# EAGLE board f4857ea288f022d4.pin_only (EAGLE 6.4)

Size 68.58 x 53.34 mm. Coordinates in mm from the lower left corner, seen from the top.
Outline: 0,0 0,53.34 64.52,53.34 66.04,51.82 66.04,40.39 68.58,37.85 68.58,5.08 66.04,2.54 66.04,0 0,0
Copper layers (1*16): Top 0.035mm / dielectric 1.5mm / Bottom 0.035mm
Design rules "pcbcart *": minimum track width 10mil, minimum drill 16mil, track to track 8mil, track to pad 8mil, pad to pad 8mil, via to via 8mil, smd to smd 8mil, copper to edge 10mil, drill to drill 8mil, minimum pad ring 10mil, minimum via ring 8mil, stop-mask expansion 4mil, vias tented up to drill 20mil, thermal gap 10mil
Holes 3.2 mm at 15.24,50.8 66.04,35.56 13.97,2.54
bRestrict: area 26.3,9.3 to 39.2,12.3

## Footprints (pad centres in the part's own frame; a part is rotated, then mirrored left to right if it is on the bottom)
SOLDERJUMPER_REFLOW_NOPASTE = smd 1.168 x 1.6: 1 -0.762,0; 2 0.762,0
0805-NO = smd 1.3 x 1.5: 1 -0.95,0; 2 0.95,0
PANASONIC_C = smd 2.6 x 1.4: + 2.05,0; - -2.05,0
1X04-CLEANBIG = drill 1.016 pad 1.778: 1 -3.81,0; 2 -1.27,0; 3 1.27,0; 4 3.81,0
1X08-CLEANBIG = drill 1.016 pad 1.778 octagon: 1 -8.89,0; 2 -6.35,0; 3 -3.81,0; 4 -1.27,0; 5 1.27,0; 6 3.81,0; 7 6.35,0; 8 8.89,0
SSOP24 = smd 0.4 x 1.25: 1 -3.575,-3.625; 2 -2.925,-3.625; 3 -2.275,-3.625; 4 -1.625,-3.625; 5 -0.975,-3.625; 6 -0.325,-3.625; 7 0.325,-3.625; 8 0.975,-3.625; 9 1.625,-3.625; 10 2.275,-3.625; 11 2.925,-3.625; 12 3.575,-3.625; 13 3.575,3.625; 14 2.925,3.625; 15 2.275,3.625; 16 1.625,3.625; 17 0.975,3.625; 18 0.325,3.625; 19 -0.325,3.625; 20 -0.975,3.625; 21 -1.625,3.625; 22 -2.275,3.625; 23 -2.925,3.625; 24 -3.575,3.625
1X05-3.5MM = drill 1 pad 2.184: 1 7,0; 2 3.5,0; 3 0,0; 4 -3.5,0; 5 -7,0
1X04_ROUND_76 = drill 1 pad 1.93 square: 1 -3.81,0 | drill 1 pad 1.93: 2 -1.27,0; 3 1.27,0; 4 3.81,0
1X10_ROUND70 = drill 1 pad 1.778 square: 1 -11.43,0 | drill 1 pad 1.778: 2 -8.89,0; 3 -6.35,0; 4 -3.81,0; 5 -1.27,0; 6 1.27,0; 7 3.81,0; 8 6.35,0; 9 8.89,0; 10 11.43,0
1X02_ROUND = drill 1 pad 1.778: 1 -1.27,0; 2 1.27,0
CHIPLED_0805_NOOUTLINE = smd 1.2 x 1.2: A 0,-1.05; C 0,1.05
1X2-3.5MM = drill 1 pad 2.184: 1 1.8,0; 2 -1.7,0
JP1 = drill 0.914 long: 1 0,-1.27; 2 0,1.27
D-PAK_TO252AA = smd 1 x 1.6: 1 -2.28,-4.8; 3 2.28,-4.8 | smd 5.4 x 6.2: 4 0,2.5
1X03 = drill 1.016: 1 -2.54,0; 2 0,0; 3 2.54,0
SOLDERJUMPER_2WAY_OPEN_NOPASTE = smd 1.168 x 1.6: 1 -1.397,0; 2 0,0; 3 1.397,0
EVQ-Q2 = smd 3.2 x 1.2: A -3.4,-2; A' 3.4,-2; B -3.4,2; B' 3.4,2
TESTPOINT_ROUND_2MM = smd 2 x 2: P$1 0,0
TSSOP28 = smd 0.305 x 0.991: 1 -4.225,-2.918; 2 -3.575,-2.918; 3 -2.925,-2.918; 4 -2.275,-2.918; 5 -1.625,-2.918; 6 -0.975,-2.918; 7 -0.325,-2.918; 8 0.325,-2.918; 9 0.975,-2.918; 10 1.625,-2.918; 11 2.275,-2.918; 12 2.925,-2.918; 13 3.575,-2.918; 14 4.225,-2.918; 15 4.225,2.918; 16 3.575,2.918; 17 2.925,2.918; 18 2.275,2.918; 19 1.625,2.918; 20 0.975,2.918; 21 0.325,2.918; 22 -0.325,2.918; 23 -0.975,2.918; 24 -1.625,2.918; 25 -2.275,2.918; 26 -2.925,2.918; 27 -3.575,2.918; 28 -4.225,2.918
ARDUINOR3_ICSP = drill 1 pad 1.676 octagon: 3V 35.56,2.54; 5V 38.1,2.54; A0 50.8,2.54; A1 53.34,2.54; A2 55.88,2.54; A3 58.42,2.54; A4 60.96,2.54; A5 63.5,2.54; AREF 23.876,50.8; D0 63.5,50.8; D1 60.96,50.8; D2 58.42,50.8; D3 55.88,50.8; D4 53.34,50.8; D5 50.8,50.8; D6 48.26,50.8; D7 45.72,50.8; D8 41.656,50.8; D9 39.116,50.8; D10 36.576,50.8; D11 34.036,50.8; D12 31.496,50.8; D13 28.956,50.8; GND 26.416,50.8; GND@1 43.18,2.54; GND@2 40.64,2.54; IOREF 30.48,2.54; RESERVED 27.94,2.54; RESET 33.02,2.54; SCL 18.796,50.8; SDA 21.336,50.8; VIN 45.72,2.54 | drill 1 pad 1.778 octagon: 5V_ICSP 66.167,30.48; GND@3 66.167,25.4; MOSI 66.167,27.94; RESET_ICSP 63.627,25.4; SCK 63.627,27.94 | drill 1 pad 1.778 square: MISO 63.627,30.48
FIDUCIAL_1MM = smd 1 x 1: 1 0,0

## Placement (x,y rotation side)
A0  [SOLDERJUMPER_REFLOW_NOPASTE]  38.1,10.79 90 top
A1  [SOLDERJUMPER_REFLOW_NOPASTE]  35.56,10.79 90 top
A2  [SOLDERJUMPER_REFLOW_NOPASTE]  33.02,10.79 90 top
A3  [SOLDERJUMPER_REFLOW_NOPASTE]  30.48,10.79 270 top
A4  [SOLDERJUMPER_REFLOW_NOPASTE]  27.69,10.79 270 top
C1  0.1uF  [0805-NO]  23.62,20.07 180 top
C2  0.1uF  [0805-NO]  24.51,23.88 0 top
C3  0.1uF  [0805-NO]  46.61,14.61 180 top
C4  47uF/16v  [PANASONIC_C]  48.39,21.72 0 top
C5  47uF+/16v  [PANASONIC_C]  13.72,15.37 0 top
C6  10uF  [0805-NO]  19.68,17.91 0 top
C9  10\0uF 6.3V  [PANASONIC_C]  7.37,42.04 180 top
C10  10uF  [0805-NO]  47.37,10.29 180 top
CN1  1X4-CLEANBIG  [1X04-CLEANBIG]  54.61,5.97 180 top
D0-7  [1X08-CLEANBIG]  54.61,47.24 180 top
IC1  TB6612FNG  [SSOP24]  13.97,22.99 270 top
IC3  TB6612FNG  [SSOP24]  54.36,14.86 90 top
J1  1X5  [1X05-3.5MM]  3.81,22.86 270 top
J2  1X5  [1X05-3.5MM]  65.15,14.22 270 top
JP1  [1X04_ROUND_76]  60.96,39.37 90 top
JP2  [1X08-CLEANBIG]  36.83,5.97 180 top
JP3  [1X10_ROUND70]  30.23,47.24 0 top
JP4  [1X02_ROUND]  57.15,9.14 180 top
LED1  Green  [CHIPLED_0805_NOOUTLINE]  15.37,10.29 270 top
MPOWER  1X2-3.5MM  [1X2-3.5MM]  20.45,3.94 0 top
PWR  [JP1]  21.84,10.16 270 top
Q1  AOD417  [D-PAK_TO252AA]  6.35,8.38 90 top
R1  10k  [0805-NO]  38.1,15.24 270 top
R2  10k  [0805-NO]  35.56,15.24 270 top
R3  10k  [0805-NO]  33.02,15.24 270 top
R4  1K  [0805-NO]  19.56,15.37 180 top
R5  10k  [0805-NO]  30.48,15.24 270 top
R6  10k  [0805-NO]  27.69,15.24 270 top
R7  10K  [0805-NO]  20.07,45.21 180 top
R8  10K  [0805-NO]  15.37,45.72 180 top
SERPWR  1X2-3.5MM  [1X2-3.5MM]  2.03,48.77 270 top
SERVO1  [1X03]  9.4,50.16 0 top
SERVO2  [1X03]  9.4,47.62 0 top
SJ1  [SOLDERJUMPER_2WAY_OPEN_NOPASTE]  36.83,8.13 180 top
SW1  SPST_TACT-EVQQ2  [EVQ-Q2]  5.46,35.94 180 top
TP1  [TESTPOINT_ROUND_2MM]  27.69,10.79 0 bottom
TP2  [TESTPOINT_ROUND_2MM]  30.48,10.79 270 bottom
TP3  [TESTPOINT_ROUND_2MM]  33.02,10.79 0 bottom
TP4  [TESTPOINT_ROUND_2MM]  35.56,10.79 0 bottom
TP5  [TESTPOINT_ROUND_2MM]  38.1,10.79 0 bottom
U2  PCA9685  [TSSOP28]  34.8,22.61 90 top
U$1  ARDUINO_R3_ICSP  [ARDUINOR3_ICSP]  0,0 0 top
U$2  FIDUCIAL  [FIDUCIAL_1MM]  48.39,1.65 0 top
U$3  FIDUCIAL  [FIDUCIAL_1MM]  1.52,43.69 0 top
U$4  FIDUCIAL  [FIDUCIAL_1MM]  65.28,38.86 0 top
U$5  [ADAFRUIT_TEXT_30MM]  55.12,12.7 0 bottom
U$6  [ADAFRUIT_3.5MM]  40.39,10.92 0 top

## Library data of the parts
A0 A1-A4 C1-C6 C10 JP1 JP3 JP4 LED1 R1-R8 SJ1 TP1-TP5 U2 U$5 U$6 = microbuilder
C9 CN1 D0-7 IC1 IC3 J1 J2 JP2 MPOWER SERPWR SERVO1 SERVO2 SW1 U$1-U$4 = adafruit
PWR = jumper
Q1 = transistor-power

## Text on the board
tPlace: Servo 1 | Opt | Servo | Servo 2 | Servo pins | S1 | S2 | PWMs | #15 | Reset | #14 | #1 | #0 | M1 | Adafruit Motor Shield v2.3 | 2 steppers or | 4 DC motors | 1.2A per motor | (3A max) | GND | M4 | M2 | VIN | GND | Jumper | Power | logic: | 3v | 5v | 4 | 5 | M3 | + | - | 5-12V Motor | Power
bPlace: For opt. servo | pwr supply cut trace | Adafruit Motor Shield v2! / Control 4 DC Motors or / 2 Stepper motors via I2C / Pins used: SDA, SCL & / A4 tied to SDA, A5 to SCL

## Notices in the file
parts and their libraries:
microbuilder: This work is placed in the public domain, and may be freely used for commercial and non-commercial work with the following conditions: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
